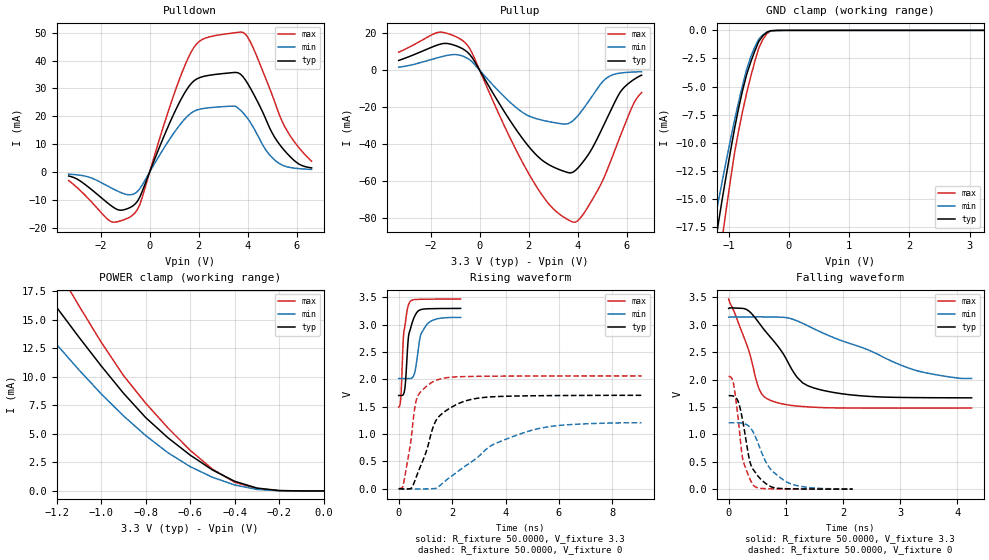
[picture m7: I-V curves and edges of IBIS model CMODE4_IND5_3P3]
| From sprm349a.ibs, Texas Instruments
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|   Model Cell CMODE4_IND5_3P3
|CMODE4_IND5_3P3
[Model]   CMODE4_IND5_3P3
Model_type   I/O
Polarity   Non-Inverting
Enable   Active-Low
Vinl =  0.8V
Vinh =  2V
Cref =  15.0000pF
Rref =  100.0000M
Vref =  0V
Vmeas =  1.65
C_comp   1.705749p   1.660791p   1.75003p
[Model Spec]
Vinl   0.8V   0.8V   0.8V
Vinh   2V   2V   2V
[Temperature Range]   25   125   -40
[Voltage Range]   3.3   3.14   3.47
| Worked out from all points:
|   slope of the pulldown table from 0 to 0.495 V, typ, clamps not added: 45.1 ohm
|   slope of the pullup table from 0 to 0.495 V, typ, clamps not added: 43.8 ohm
|   GND clamp passes 1 mA (typ) near -0.50 V on its own axis
|   POWER clamp passes 1 mA (typ) near -0.42 V on its own axis
|   rising waveform, R_fixture 50.0000, V_fixture 3.3: 20-80 % time 205ps typ, 283ps min, 156ps max; typ from 1.71 V to 3.3 V
|   rising waveform, R_fixture 50.0000, V_fixture 0: 20-80 % time 852ps typ, 2.32ns min, 381ps max; typ from 0 V to 1.71 V
|   falling waveform, R_fixture 50.0000, V_fixture 3.3: 20-80 % time 669ps typ, 1.55ns min, 358ps max; typ from 3.3 V to 1.67 V
|   falling waveform, R_fixture 50.0000, V_fixture 0: 20-80 % time 217ps typ, 399ps min, 163ps max; typ from 1.71 V to 0.002 V
[POWER_clamp]
|   voltage   I(typ)   I(min)   I(max)
-3.3V     84.32mA    63.21mA    102.6mA
-1.4V     21.7mA     17.52mA    26.35mA
-1.367V   20.74mA    16.73mA    25.21mA
-1.233V   17.01mA    13.62mA    20.69mA
-1.133V   14.37mA    11.37mA    17.36mA
-900mV    8.579mA    6.593mA    10.13mA
-800mV    6.436mA    4.86mA     7.699mA
-600mV    3.143mA    2.131mA    3.565mA
-500mV    1.84mA     1.2mA      1.913mA
-400mV    844.9uA    518.8uA    757.6uA
-300mV    251.4uA    131.2uA    193.7uA
0V        112.2nA    201.8nA    235.2nA
[Pulldown]
|   voltage   I(typ)   I(min)   I(max)
-3.3V     -1.414mA   -745.4uA   -3.05mA
-1.6V     -11.86mA   -5.525mA   -17.66mA
-700mV    -12.23mA   -8.019mA   -15.5mA
-400mV    -8.953mA   -5.978mA   -11.65mA
900mV     19.24mA    12.9mA     25.53mA
1.7V      31.81mA    21.22mA    43.17mA
2.2V      34.3mA     22.8mA     47.78mA
3.7V      35.12mA    22.19mA    50.19mA
4.1V      30.16mA    17.85mA    46.74mA
5.1V      12.38mA    4.294mA    25.08mA
5.7V      5.756mA    1.687mA    13.38mA
6.6V      1.491mA    938uA      3.886mA
[Pullup]
|   voltage   I(typ)   I(min)   I(max)
-3.3V     5.279mA    1.68mA     9.743mA
-1.7V     13.72mA    6.799mA    20.48mA
-600mV    10.83mA    7.151mA    14.99mA
1.3V      -28.42mA   -18.04mA   -38.22mA
2.2V      -44.3mA    -25.71mA   -60.41mA
3V        -52.29mA   -28.23mA   -74.9mA
3.8V      -55.14mA   -27.3mA    -82.11mA
4.3V      -48.01mA   -19.44mA   -76.32mA
5.2V      -25.74mA   -3.981mA   -53.86mA
5.8V      -10.57mA   -1.414mA   -33.26mA
6.3V      -4.87mA    -940.5uA   -17.38mA
6.6V      -2.661mA   -794.2uA   -12.11mA
[GND_clamp]
|   voltage   I(typ)   I(min)   I(max)
-3.3V     -100.4mA   -76.62mA   -119.8mA
-1.3V     -21.74mA   -18.91mA   -26.19mA
-1.233V   -19.35mA   -17.01mA   -23.53mA
-1.167V   -17.04mA   -15.12mA   -20.89mA
-1.1V     -14.82mA   -13.26mA   -18.27mA
-1.033V   -12.73mA   -11.45mA   -15.71mA
-900mV    -8.706mA   -7.949mA   -10.85mA
-700mV    -3.917mA   -3.459mA   -5.57mA
-500mV    -997.2uA   -790.2uA   -1.589mA
-366.7mV  -173.2uA   -169.7uA   -302.5uA
-166.7mV  -4.979uA   -6.05uA    -6.593uA
3.233V    80.05nA    2.439uA    205.4nA
[Ramp]
| variable   typ   min   max
dV/dt_f  0.9852839/0.6660964n  0.7326518/1.728273n   1.200995/0.3597556n
dV/dt_r   1.031415/0.8564381n  0.7444951/2.445132n   1.243503/0.3800221n
R_load = 50
[Rising Waveform]
R_fixture = 50.0000
V_fixture = 3.3
V_fixture_min = 3.14
V_fixture_max = 3.47
|   time   V(typ)   V(min)   V(max)
0s        1.706V     2.016V     1.495V
80ps      1.706V     2.017V     1.664V
168ps     1.719V     2.017V     2.691V
224ps     1.81V      2.017V     2.946V
352ps     2.703V     2.016V     3.339V
408ps     2.875V     2.016V     3.409V
576ps     3.131V     2.084V     3.458V
808ps     3.272V     2.782V     3.464V
1.04ns    3.29V      2.995V     3.466V
2.32ns    3.298V     3.134V     3.469V
[Rising Waveform]
R_fixture = 50.0000
V_fixture = 0
V_fixture_min = 0
V_fixture_max = 0
|   time   V(typ)   V(min)   V(max)
0s        39.15uV    23.94uV    60.36uV
136ps     -2.38mV    31.36uV    17.34mV
200ps     -6.39mV    30.06uV    140.7mV
488ps     20.72mV    -1.313mV   996mV
664ps     222.7mV    -4.67mV    1.63V
1.36ns    1.213V     4.272mV    1.976V
2.552ns   1.614V     434mV      2.053V
3.504ns   1.682V     800.6mV    2.059V
4.728ns   1.699V     1.033V     2.061V
9.096ns   1.709V     1.206V     2.064V
[Falling Waveform]
R_fixture = 50.0000
V_fixture = 3.3
V_fixture_min = 3.14
V_fixture_max = 3.47
|   time   V(typ)   V(min)   V(max)
0s        3.3V       3.14V      3.47V
352ps     3.252V     3.145V     2.529V
536ps     3.027V     3.145V     1.817V
712ps     2.797V     3.143V     1.63V
920ps     2.524V     3.139V     1.562V
1.2ns     2.038V     3.071V     1.518V
1.48ns    1.851V     2.932V     1.497V
2.224ns   1.713V     2.624V     1.481V
3.208ns   1.672V     2.189V     1.48V
4.248ns   1.668V     2.022V     1.481V
[Falling Waveform]
R_fixture = 50.0000
V_fixture = 0
V_fixture_min = 0
V_fixture_max = 0
|   time   V(typ)   V(min)   V(max)
0s        1.707V     1.212V     2.062V
88ps      1.696V     1.213V     1.907V
176ps     1.572V     1.212V     1.198V
224ps     1.364V     1.206V     706.7mV
256ps     1.19V      1.2V       504mV
368ps     517.2mV    1.134V     196.7mV
456ps     320.8mV    985.5mV    49.78mV
704ps     65.32mV    405.7mV    8.428mV
1.016ns   8.885mV    131.1mV    3.709mV
2.168ns   2.345mV    6.414mV    871.5uV
